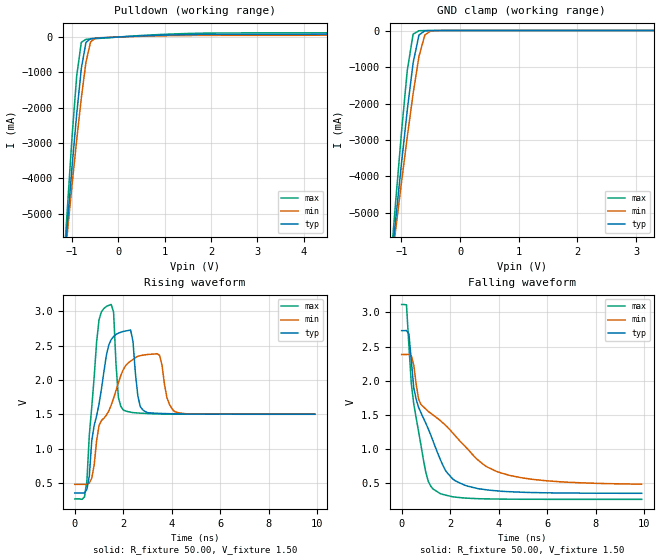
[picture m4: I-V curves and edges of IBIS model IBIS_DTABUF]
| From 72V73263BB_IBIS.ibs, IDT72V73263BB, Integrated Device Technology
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|   Model IBIS_DTABUF
[Model]   IBIS_DTABUF
Model_type   I/O_open_drain
Polarity   Non-Inverting
Enable   Active-High
Vinl =  0.000V
Vinh =  3.300V
Vmeas =  1.500V
Cref = 30.000pF
Rref = 50.000
Vref =  1.500V
C_comp   3.00pF   2.00pF   4.00pF
[Temperature Range]   25.00   85.00   -40.00
[Voltage Range]   3.30V   3.00V   3.60V
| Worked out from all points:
|   slope of the pulldown table from 0 to 0.495 V, typ, clamps not added: 16.1 ohm
|   GND clamp passes 1 mA (typ) near -0.51 V on its own axis
|   rising waveform, R_fixture 50.00, V_fixture 1.50: 20-80 % time 180ps typ, 223ps min, 120ps max; typ from 0.355 V to 1.5 V
|   falling waveform, R_fixture 50.00, V_fixture 1.50: 20-80 % time 1.21ns typ, 2.49ns min, 608ps max; typ from 2.73 V to 0.356 V
[Pulldown]
| voltage   I(typ)   I(min)   I(max)
-3.3V     -42.01A    -36.04A    -50.9A
-1.5V     -11.71A    -10.89A    -12.87A
-1V       -3.67A     -4.184A    -2.828A
-900mV    -2.19A     -2.919A    -1.111A
-800mV    -893.8mA   -1.729A    -150.1mA
-700mV    -151.7mA   -712.3mA   -66.27mA
-600mV    -46.32mA   -137.9mA   -55.05mA
-500mV    -34.57mA   -33.69mA   -46mA
-400mV    -27.67mA   -20.5mA    -37.18mA
1.5V      67.91mA    43.34mA    99.95mA
4.7V      84.5mA     56.12mA    122mA
6.6V      131mA      78.82mA    191mA
[GND_clamp]
| voltage   I(typ)   I(min)   I(max)
-3.3V     -42.01A    -36.04A    -50.9A
-1.2V     -6.817A    -6.818A    -6.727A
-1.1V     -5.222A    -5.488A    -4.737A
-1V       -3.667A    -4.183A    -2.82A
-900mV    -2.185A    -2.917A    -1.095A
-800mV    -883mA     -1.726A    -98.49mA
-700mV    -122mA     -706mA     -5.285mA
-600mV    -7.89mA    -122mA     -799uA
-500mV    -309uA     -12.24mA   -81.59uA
3.3V      3.324nA    12.74nA    3.301nA
[Ramp]
| variable   typ   min   max
dV/dt_r   1.46/0.21n   1.13/0.23n   1.74/0.17n
dV/dt_f   1.46/1.39n   1.11/2.65n   1.74/0.72n
R_load = 50.00
[Rising Waveform]
R_fixture = 50.00
V_fixture = 1.50
C_fixture = 0.000F
| time   V(typ)   V(min)   V(max)
0s        355mV      480mV      268mV
400ps     355mV      480mV      298mV
1ns       1.65V      1.335V     2.877V
1.4ns     2.506V     1.546V     3.085V
1.6ns     2.631V     1.733V     2.989V
1.8ns     2.68V      1.96V      1.74V
2ns       2.705V     2.15V      1.562V
3ns       1.522V     2.369V     1.51V
4.2ns     1.506V     1.528V     1.501V
9.9ns     1.5V       1.5V       1.5V
[Falling Waveform]
R_fixture = 50.00
V_fixture = 1.50
C_fixture = 0.000F
| time   V(typ)   V(min)   V(max)
0s        2.732V     2.384V     3.114V
200ps     2.735V     2.383V     3.108V
300ps     2.682V     2.386V     2.502V
500ps     1.894V     2.229V     1.659V
700ps     1.609V     1.728V     1.255V
1.3ns     1.114V     1.499V     417mV
1.9ns     647mV      1.318V     322mV
2.7ns     462mV      1.011V     285mV
4.5ns     379mV      614mV      270mV
9.9ns     356mV      489mV      268mV
